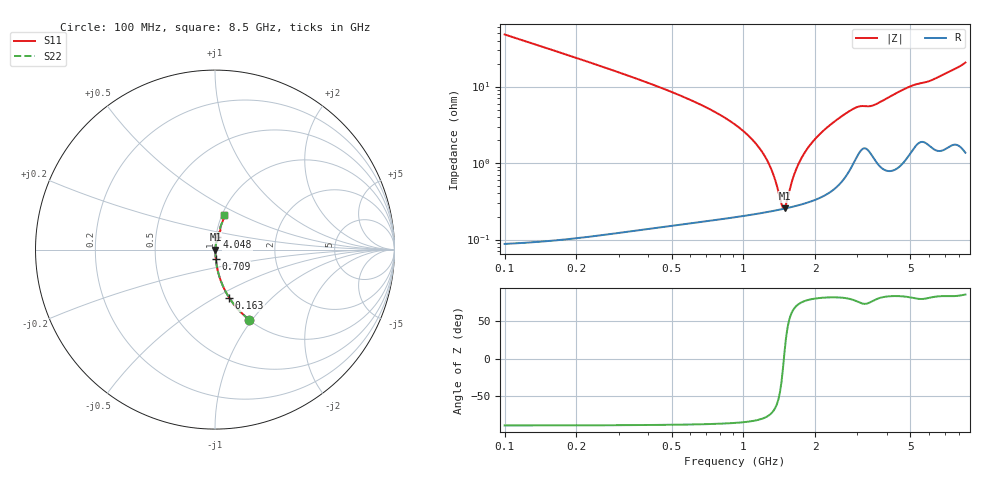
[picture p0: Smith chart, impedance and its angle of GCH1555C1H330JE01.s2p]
!Murata Part Number: GCH1555C1H330JE01
!These Parameters are Measured in Series Mode Connection
!Data Generated on Mar 13, 2026
!  o--ll--o
!Port1  Port2
!  o------o
!Operation Temp=25[degC], DC Bias Voltage=0[V]
!Freq. Start=100[MHz] Stop=9[GHz] 401[Steps]
# Hz S RI R 50
!Freq.(Hz) S11(Real) S11(Imag) S21(Real) S21(Imag) S12(Real) S12(Imag) S22(Real) S22(Imag)
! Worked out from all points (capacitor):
!   401 points, 100 MHz to 8.5 GHz, reference 50 ohm
!   read as one part in series: C = 33 pF near 142 MHz
!   lowest |Z| = 257 mohm at 1.486 GHz (marker M1)
!   series resonance near 1.477 GHz, so ESL is about 350 pH
!   S11 on the Smith chart (normalised r, x): 100 MHz: 1.00, -0.96; 163 MHz: 1.00, -0.58; 709 MHz: 1.00, -0.10; 4.048 GHz: 1.02, +0.14; 8.5 GHz: 1.03, +0.41
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1e8  0.1876 -0.3895  0.8124 0.3895  0.8124 0.3895  0.1876 -0.3895
1.63e8  0.0793 -0.2686  0.9207 0.2686  0.9207 0.2686  0.0793 -0.2686
3.52e8  0.0176 -0.1264  0.9824 0.1264  0.9824 0.1264  0.0176 -0.1264
7.09e8  0.00444 -0.0518  0.9956 0.0518  0.9956 0.0518  0.00444 -0.0518
9.82e8  0.00275 -0.0272  0.9972 0.0272  0.9972 0.0272  0.00275 -0.0272
1.171e9  0.00243 -0.0152  0.9976 0.0152  0.9976 0.0152  0.00243 -0.0152
1.318e9  0.0024 -0.00743  0.9976 0.00743  0.9976 0.00743  0.0024 -0.00743
1.444e9  0.00248 -0.00148  0.9975 0.00148  0.9975 0.00148  0.00248 -0.00148
1.486e9  0.00253 0.000391  0.9975 -0.000391  0.9975 -0.000391  0.00253 0.000391
1.507e9  0.00256 0.00131  0.9974 -0.00131  0.9974 -0.00131  0.00256 0.00131
1.612e9  0.00272 0.00573  0.9973 -0.00573  0.9973 -0.00573  0.00272 0.00573
1.675e9  0.00283 0.00826  0.9972 -0.00826  0.9972 -0.00826  0.00283 0.00826
1.78e9  0.00307 0.0123  0.9969 -0.0123  0.9969 -0.0123  0.00307 0.0123
1.927e9  0.00347 0.0178  0.9965 -0.0178  0.9965 -0.0178  0.00347 0.0178
2.326e9  0.00522 0.0316  0.9948 -0.0316  0.9948 -0.0316  0.00522 0.0316
2.914e9  0.0128 0.0498  0.9872 -0.0498  0.9872 -0.0498  0.0128 0.0498
3.46e9  0.0151 0.0533  0.9849 -0.0533  0.9849 -0.0533  0.0151 0.0533
4.048e9  0.0128 0.0703  0.9872 -0.0703  0.9872 -0.0703  0.0128 0.0703
4.3e9  0.0142 0.0779  0.9858 -0.0779  0.9858 -0.0779  0.0142 0.0779
5.707e9  0.0299 0.1058  0.9701 -0.1058  0.9701 -0.1058  0.0299 0.1058
7.114e9  0.0368 0.1435  0.9632 -0.1435  0.9632 -0.1435  0.0368 0.1435
8.5e9  0.0524 0.1922  0.9476 -0.1922  0.9476 -0.1922  0.0524 0.1922
